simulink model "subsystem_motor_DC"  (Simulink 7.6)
settings: Solver=ode45  StartTime=0.0  StopTime=10.0  RelTol=1e-3
libraries: fl_lib x8, nesl_utility x3

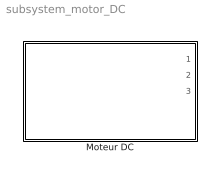
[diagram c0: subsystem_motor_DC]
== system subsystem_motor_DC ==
  Moteur DC : Subsystem

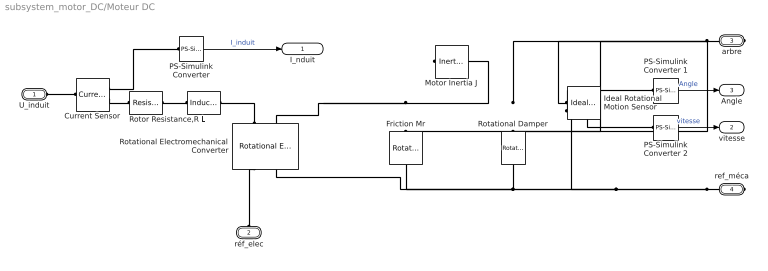
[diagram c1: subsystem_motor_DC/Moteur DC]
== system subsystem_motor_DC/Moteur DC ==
  Current Sensor : fl_lib/Electrical/Electrical Sensors/Current Sensor  DialogController=NetworkEngine.DynNeDlgSource  SystemSampleTime=-1  i1_Log=off  v1_Log=off  LocalVarNames=|i1|v1  LocalVarDescs=|i1|v1  LocalVarLogging=[0 0]
  Friction Mr : fl_lib/Mechanical/Rotational Elements/Rotational Friction  DialogController=NetworkEngine.DynNeDlgSource  SystemSampleTime=-1  brkwy_trq=0.02e-3 N*m  Col_trq=0.02e-3 N*m  visc_coef=0 N*m/(rad/s)  trans_coef=10 s/rad  vel_thr=0.1 rad/s  t_Log=off  w_Log=off  LocalVarNames=|friction_torque|rel_velocity|power  LocalVarDescs=|Friction torque (N*m)|Relative velocity (rad/s)|Power (W)  LocalVarLogging=[0 0 0]
  Ideal Rotational Motion Sensor : fl_lib/Mechanical/Mechanical Sensors/Ideal Rotational Motion Sensor  DialogController=NetworkEngine.DynNeDlgSource  SystemSampleTime=-1  offset=0 rad  w_Log=off  t_Log=off  phi_Log=off  LocalVarNames=|w|t|phi  LocalVarDescs=|w|t|phi  LocalVarLogging=[]
  L : fl_lib/Electrical/Electrical Elements/Inductor  DialogController=NetworkEngine.DynNeDlgSource  SystemSampleTime=-1  l=12e-6 H  i0=0 A  r=0 Ohm  g=1e-09 1/Ohm  i_Log=off  v_Log=off  i_L_Log=off  LocalVarNames=|current|voltage|power  LocalVarDescs=|Inductor current (A) |Voltage across inductor (V)|Power (W)  LocalVarLogging=[0 0 0]
  Motor Inertia J : fl_lib/Mechanical/Rotational Elements/Inertia  DialogController=NetworkEngine.DynNeDlgSource  SystemSampleTime=-1  inertia=0.01 g*cm^2  initial_velocity=0 rad/s  t_Log=off  LocalVarNames=|torque|velocity  LocalVarDescs=|Inertia torque (N*m)|Inertia absolute velocity (rad/s)  LocalVarLogging=[0 0]
  PS-Simulink Converter : nesl_utility/PS-Simulink Converter  DialogController=NetworkEngine.DynNeUtilDlgSource  SystemSampleTime=-1  PhysicalDomain=network_engine_domain  LeftPortType=input  RightPortType=output  SubClassName=ps_output  Unit=1  AffineConversion=off
  PS-Simulink Converter 1 : nesl_utility/PS-Simulink Converter  DialogController=NetworkEngine.DynNeUtilDlgSource  SystemSampleTime=-1  PhysicalDomain=network_engine_domain  LeftPortType=input  RightPortType=output  SubClassName=ps_output  Unit=rpm  AffineConversion=off
  PS-Simulink Converter 2 : nesl_utility/PS-Simulink Converter  DialogController=NetworkEngine.DynNeUtilDlgSource  SystemSampleTime=-1  PhysicalDomain=network_engine_domain  LeftPortType=input  RightPortType=output  SubClassName=ps_output  Unit=rpm  AffineConversion=off
  Rotational Electromechanical Converter : fl_lib/Electrical/Electrical Elements/Rotational Electromechanical Converter  DialogController=NetworkEngine.DynNeDlgSource  SystemSampleTime=-1  K=0.072e-3*60/(2*pi) V/(rad/s)  i_Log=off  v_Log=off  t_Log=off  w_Log=off  LocalVarNames=|current|voltage|power|torque|speed  LocalVarDescs=|Current (A)|Voltage (V)|Power (W)|Torque (Nm)|Angular speed (rad/s)  LocalVarLogging=[0 0 0 0 0]
  Rotational Damper : fl_lib/Mechanical/Rotational Elements/Rotational Damper  DialogController=NetworkEngine.DynNeDlgSource  SystemSampleTime=-1  D=0.001 N*m/(rad/s)  t_Log=off  w_Log=off  LocalVarNames=|t|w  LocalVarDescs=|t|w  LocalVarLogging=[0 0]
  Rotor Resistance,R : fl_lib/Electrical/Electrical Elements/Resistor  Tag=Factory Generic  DialogController=NetworkEngine.DynNeDlgSource  SystemSampleTime=-1  R=3.9 Ohm  i_Log=off  v_Log=off  LocalVarNames=|current|voltage|power  LocalVarDescs=|Resistor current (A)|Voltage across resistor (V)|Power (W)  LocalVarLogging=[0 0 0]
  U_induit : PMIOPort  Port=1  Side=Left
  réf_elec : PMIOPort  Port=2  Side=Left
  arbre : PMIOPort  Port=3  Side=Right
  ref_méca : PMIOPort  Port=4  Side=Right
  I_nduit : Outport
  vitesse : Outport  Port=2
  Angle : Outport  Port=3
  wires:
  PS-Simulink Converter/1 -> I_nduit/1  "I_induit"
  PS-Simulink Converter 1/1 -> Angle/1  "Angle"
  PS-Simulink Converter 2/1 -> vitesse/1  "vitesse"
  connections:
  Current Sensor/RConn1 -- PS-Simulink Converter/LConn1
  Current Sensor/RConn2 -- Rotor Resistance,R/LConn1
  arbre/RConn1 -- Motor Inertia J/LConn1 -- Rotational Electromechanical Converter/LConn2 -- Friction Mr/LConn1 -- Rotational Damper/LConn1 -- Ideal Rotational Motion Sensor/LConn1
  ref_méca/RConn1 -- Friction Mr/RConn1 -- Rotational Electromechanical Converter/RConn2 -- Rotational Damper/RConn1 -- Ideal Rotational Motion Sensor/RConn1
  Ideal Rotational Motion Sensor/RConn2 -- PS-Simulink Converter 2/LConn1
  Ideal Rotational Motion Sensor/RConn3 -- PS-Simulink Converter 1/LConn1
  L/LConn1 -- Rotor Resistance,R/RConn1
  Rotational Electromechanical Converter/LConn1 -- L/RConn1
  U_induit/RConn1 -- Current Sensor/LConn1
  réf_elec/RConn1 -- Rotational Electromechanical Converter/RConn1
